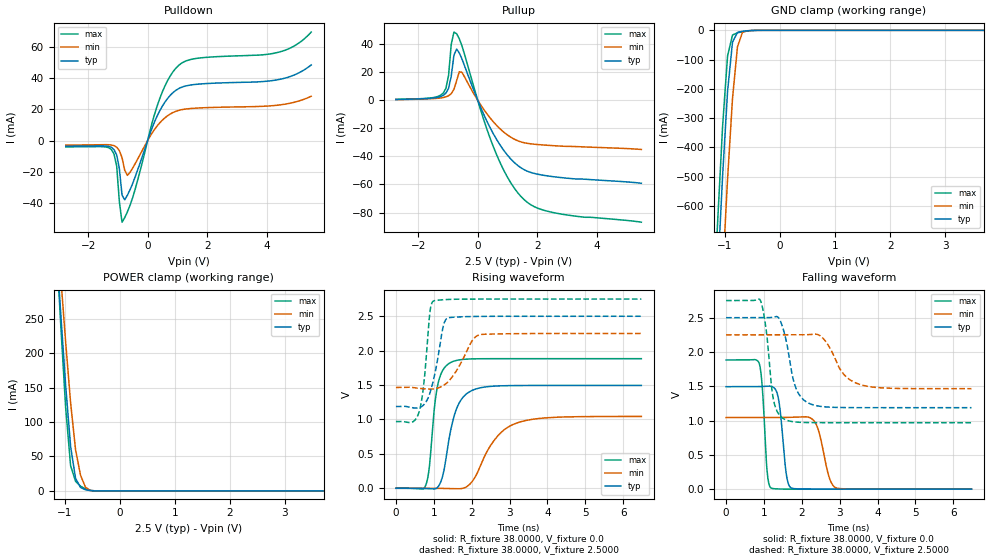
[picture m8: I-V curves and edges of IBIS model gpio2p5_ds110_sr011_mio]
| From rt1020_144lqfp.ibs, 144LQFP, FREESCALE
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[Model] gpio2p5_ds110_sr011_mio
|   Model gpio2p5_ds110_sr011_mio
| This model was characterised for following simulation conditions:
| External (pad) voltage:
|   - Typ: 2.5V,   - Min: 2.25V,   - Max: 2.75V
| Library cells for typ/min/max conditions are connected as defined below:
|  pad - External Pad
|  ipp_do - Core Input
|  ipp_obe - Output Buffer Enable
|  esd_boost - ovdd
|  ipp_dse0 - vssi
|  ipp_dse1 - vddi
|  ipp_dse2 - vddi
|  ipp_fsel0 - vddi
|  ipp_fsel1 - vddi
|  ipp_ina - ipp_ina
|  ipp_ind - ipp_ind
|  ipp_pwr_stable - vddi
|  ipp_sre - vssi
|  ovdd - ovdd
|  ovss - ovss
|  vddi - vddi
|  vssi - vssi
| All other pins connected to ground
Model_type I/O
Polarity   Non-Inverting
Enable   Active-High
Vinl =   0.7500V
Vinh =   1.7500V
Vmeas =  1.2500V
Cref =   0.0F
Rref =   38.0000
Vref =   1.2500V
C_comp   1.2356pF   1.1994pF   1.2834pF
|C_comp_pullup   0.6222pF   0.6389pF   0.6073pF
|C_comp_pulldown   0.5474pF   0.5788pF   0.5258pF
[Model Spec]
| variable   typ   min   max
Vinh   1.7500V   1.5750V   1.9250V
Vinl   0.7500V   0.6750V   0.8250V
S_overshoot_high   2.5000V   2.2500V   2.7500V
S_overshoot_low   0.0V   0.0V   0.0V
Vmeas   1.2500V   1.1250V   1.3750V
Vref   1.2500V   1.1250V   1.3750V
Cref   0.0F   0.0F   0.0F
Rref   38.0000   38.0000   38.0000
[Temperature Range]   25.0000   0.1050k   -20.0000
[Voltage Range]   2.5000V   2.2500V   2.7500V
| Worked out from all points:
|   slope of the pulldown table from 0 to 0.375 V, typ, clamps not added: 21 ohm
|   slope of the pullup table from 0 to 0.375 V, typ, clamps not added: 21.1 ohm
|   GND clamp passes 1 mA (typ) near -0.54 V on its own axis
|   POWER clamp passes 1 mA (typ) near -0.57 V on its own axis
|   rising waveform, R_fixture 38.0000, V_fixture 0.0: 20-80 % time 349ps typ, 692ps min, 211ps max; typ from 0 V to 1.49 V
|   rising waveform, R_fixture 38.0000, V_fixture 2.5000: 20-80 % time 273ps typ, 466ps min, 175ps max; typ from 1.19 V to 2.5 V
|   falling waveform, R_fixture 38.0000, V_fixture 0.0: 20-80 % time 154ps typ, 252ps min, 114ps max; typ from 1.49 V to 0 V
|   falling waveform, R_fixture 38.0000, V_fixture 2.5000: 20-80 % time 305ps typ, 503ps min, 203ps max; typ from 2.5 V to 1.19 V
[Pulldown]
|Voltage   I(typ)   I(min)   I(max)
-2.75V    -3.628mA   -2.927mA   -4.055mA
-1.22V    -4.29mA    -2.837mA   -5.71mA
-1.04V    -9.229mA   -4.254mA   -16.33mA
-950mV    -18mA      -6.412mA   -39.1mA
-860mV    -34.94mA   -10.95mA   -52.37mA
-770mV    -38.02mA   -19.05mA   -49.48mA
-680mV    -35.11mA   -22.35mA   -45.77mA
400mV     18.83mA    11.19mA    26.54mA
1.03V     33.21mA    19.29mA    48.01mA
1.66V     36.13mA    20.85mA    52.77mA
4.36V     38.98mA    22.69mA    56.49mA
5.5V      48.55mA    28.45mA    69.61mA
[Pullup]
|Voltage   I(typ)   I(min)   I(max)
-2.75V    590uA      510uA      650uA
-1.16V    3.505mA    1.949mA    5.151mA
-980mV    8.563mA    3.24mA     17.77mA
-890mV    17.3mA     4.747mA    39.95mA
-800mV    32.11mA    7.79mA     48.61mA
-710mV    36.51mA    13.91mA    47.46mA
-530mV    29.43mA    19.92mA    38.77mA
550mV     -24.83mA   -15.93mA   -34.44mA
1V        -39.13mA   -24.74mA   -54.84mA
1.54V     -49.23mA   -30.16mA   -70.43mA
2.62V     -54.66mA   -32.45mA   -80.37mA
5.5V      -59.14mA   -35.06mA   -86.89mA
[GND_clamp]
|Voltage   I(typ)   I(min)   I(max)
-2.75V    -7.488A    -7.708A    -7.379A
-1.22V    -1.193A    -1.537A    -1.012A
-1.13V    -835.6mA   -1.18A     -654.7mA
-1.04V    -497.8mA   -833mA     -328mA
-950mV    -208.9mA   -508.7mA   -87.54mA
-860mV    -39.89mA   -232.5mA   -15.89mA
-770mV    -7.264mA   -56.44mA   -8.363mA
-680mV    -3.422mA   -7.048mA   -4.851mA
-590mV    -1.552mA   -1.455mA   -2.251mA
-500mV    -482.7uA   -438.2uA   -698.4uA
5.5V      0A         0A         0A
[POWER_clamp]
|Voltage   I(typ)   I(min)   I(max)
-2.75V    2.386A     2.288A     2.687A
-1.16V    368.2mA    410.8mA    372.9mA
-1.07V    258.5mA    311.8mA    242.5mA
-980mV    153.1mA    216.2mA    121.1mA
-890mV    64.5mA     128mA      36.56mA
-800mV    18.16mA    59.6mA     13.82mA
-710mV    5.012mA    22.76mA    6.935mA
-620mV    1.706mA    5.315mA    2.959mA
-530mV    383.1uA    636.8uA    795.1uA
-440mV    42.36uA    66.97uA    84.45uA
5.5V      0A         0A         0A
[Ramp]
| variable   typ   min   max
dV/dt_r  0.8966/0.3488n   0.6265/0.6915n   1.1302/0.2108n
dV/dt_f  0.7872/0.3048n   0.4709/0.5030n   1.0685/0.2028n
R_load = 38.0000
[Rising Waveform]
R_fixture= 38.0000
V_fixture= 0.0
V_fixture_min= 0.0
V_fixture_max= 0.0
|time   V(typ)   V(min)   V(max)
0s        651.3pV    2.542nV    2.056nV
785.1ps   -3.793mV   207.2uV    39.62mV
875.5ps   -6.268mV   7.483uV    275.6mV
1.095ns   10.95mV    -1.033mV   1.478V
1.258ns   232.8mV    -2.279mV   1.733V
1.428ns   794mV      -4.309mV   1.823V
1.872ns   1.376V     24.36mV    1.877V
2.638ns   1.486V     728.3mV    1.883V
3.189ns   1.493V     948.2mV    1.884V
6.48ns    1.494V     1.044V     1.884V
[Rising Waveform]
R_fixture= 38.0000
V_fixture= 2.5000
V_fixture_min= 2.2500
V_fixture_max= 2.7500
|time   V(typ)   V(min)   V(max)
0s        1.188V     1.465V     969.2mV
429.6ps   1.171V     1.466V     961.3mV
606.4ps   1.169V     1.453V     1.099V
743ps     1.218V     1.446V     1.55V
899.1ps   1.387V     1.441V     2.566V
998.4ps   1.591V     1.444V     2.723V
1.242ns   2.338V     1.49V      2.74V
1.376ns   2.477V     1.548V     2.744V
2.194ns   2.498V     2.228V     2.75V
6.48ns    2.5V       2.25V      2.75V
[Falling Waveform]
R_fixture= 38.0000
V_fixture= 0.0
V_fixture_min= 0.0
V_fixture_max= 0.0
|time   V(typ)   V(min)   V(max)
0s        1.494V     1.044V     1.884V
876.7ps   1.495V     1.044V     1.832V
1.09ns    1.501V     1.044V     225mV
1.197ns   1.499V     1.044V     14.75mV
1.379ns   1.333V     1.044V     3.06mV
1.585ns   242.1mV    1.046V     936.1uV
1.718ns   18.4mV     1.048V     476.6uV
2.356ns   597.6uV    969.8mV    63.85uV
2.894ns   104.9uV    21.03mV    29.08uV
6.48ns    -200.2nV   7.429uV    -704.6nV
[Falling Waveform]
R_fixture= 38.0000
V_fixture= 2.5000
V_fixture_min= 2.2500
V_fixture_max= 2.7500
|time   V(typ)   V(min)   V(max)
0s        2.5V       2.25V      2.75V
902.6ps   2.5V       2.25V      2.757V
1.048ns   2.499V     2.25V      2.373V
1.249ns   2.508V     2.25V      1.312V
1.561ns   2.228V     2.25V      1.014V
1.85ns    1.466V     2.25V      978.6mV
2.257ns   1.236V     2.256V     970.3mV
2.563ns   1.202V     2.198V     969.4mV
3.544ns   1.188V     1.524V     969.3mV
6.48ns    1.188V     1.465V     969.2mV
